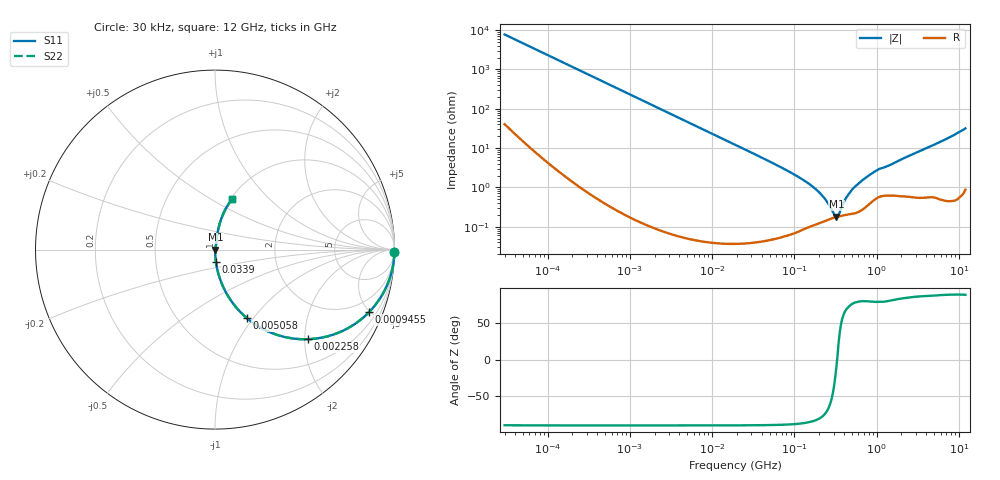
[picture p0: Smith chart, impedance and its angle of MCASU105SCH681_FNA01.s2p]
! MCASU105SCH681_FNA01  S-PARAMETER MODEL  ( General Type )
! Model Generated by TAIYO YUDEN Corporation (http://www.ty-top.com)
! Version 1.0
! TAIYO YUDEN Control No. 130207
! Copyright(c) 2013 TAIYO YUDEN CO.,LTD. All Rights Reserved.
! Product Description (link to TY-COMPAS)
! https://ds.yuden.co.jp/TYCOMPAS/or/detail?pn=MCASU105SCH681JFNA01&u=M
! Products Name : Multilayer Ceramic Capacitors
! Characteristics :
!  Capacitance : 680 pF , Rated Voltage : 50V , TCC : CH / C0H
!  Case Size : 1.0 x 0.5 / 0.039 x 0.02 [mm/inch] , Thickness : 0.5 / 0.02 [mm/inch]
!  (Conditions: Temperature = 25 degC , DC Bias Current/Voltage = 0A / 0V)
! External Node Assignments :
!  1  o---| |---o  2
! GND o---------o GND
! Frequency Range : 30000Hz  -  12GHz  [ 401 STEP ]
# MHz S RI R 50
! Freq[MHz].  S11 Real  S11 Imag  S21 Real  S21 Imag  S12 Real  S12 Imag  S22 Real  S22 Imag
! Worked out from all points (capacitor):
!   401 points, 30 kHz to 12 GHz, reference 50 ohm
!   read as one part in series: C = 682 pF near 32 kHz
!   lowest |Z| = 179 mohm at 324 MHz (marker M1)
!   series resonance near 331 MHz, so ESL is about 340 pH
!   S11 on the Smith chart (normalised r, x): 30 kHz: open; 945.5 kHz: 1.00, -4.93; 2.258 MHz: 1.00, -2.07; 5.058 MHz: 1.00, -0.92; 33.9 MHz: 1.00, -0.14; 12 GHz: 1.02, +0.63
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0.03  0.9998 -0.0129  0.000232 0.0129  0.000232 0.0129  0.9998 -0.0129
0.260295  0.9876 -0.1102  0.0124 0.1102  0.0124 0.1102  0.9876 -0.1102
0.546493  0.9478 -0.222  0.0522 0.222  0.0522 0.222  0.9478 -0.222
0.945523  0.8587 -0.348  0.1413 0.348  0.1413 0.348  0.8587 -0.348
1.437935  0.7245 -0.4464  0.2755 0.4464  0.2755 0.4464  0.7245 -0.4464
2.258455  0.5161 -0.4993  0.4839 0.4993  0.4839 0.4993  0.5161 -0.4993
5.057549  0.1756 -0.3799  0.8244 0.3799  0.8244 0.3799  0.1756 -0.3799
8.750395  0.0666 -0.2486  0.9334 0.2486  0.9334 0.2486  0.0666 -0.2486
18.97367  0.0151 -0.1206  0.9849 0.1206  0.9849 0.1206  0.0151 -0.1206
33.90345  0.00501 -0.0677  0.995 0.0677  0.995 0.0677  0.00501 -0.0677
92.13054  0.00119 -0.0233  0.9988 0.0233  0.9988 0.0233  0.00119 -0.0233
164.6252  0.00116 -0.0107  0.9988 0.0107  0.9988 0.0107  0.00116 -0.0107
227.273  0.00138 -0.00542  0.9986 0.00542  0.9986 0.00542  0.00138 -0.00542
303.8045  0.0017 -0.00123  0.9983 0.00123  0.9983 0.00123  0.0017 -0.00123
324.0443  0.00176 -0.00032  0.9982 0.00032  0.9982 0.00032  0.00176 -0.00032
345.6326  0.00182 0.000801  0.9982 -0.000801  0.9982 -0.000801  0.00182 0.000801
433.1624  0.00204 0.00534  0.998 -0.00534  0.998 -0.00534  0.00204 0.00534
542.8588  0.00229 0.0101  0.9977 -0.0101  0.9977 -0.0101  0.00229 0.0101
939.2353  0.0054 0.0243  0.9946 -0.0243  0.9946 -0.0243  0.0054 0.0243
1428.372  0.00744 0.0355  0.9926 -0.0355  0.9926 -0.0355  0.00744 0.0355
5188.566  0.0208 0.1229  0.9792 -0.1229  0.9792 -0.1229  0.0208 0.1229
12000  0.0974 0.2829  0.9026 -0.2829  0.9026 -0.2829  0.0974 0.2829
